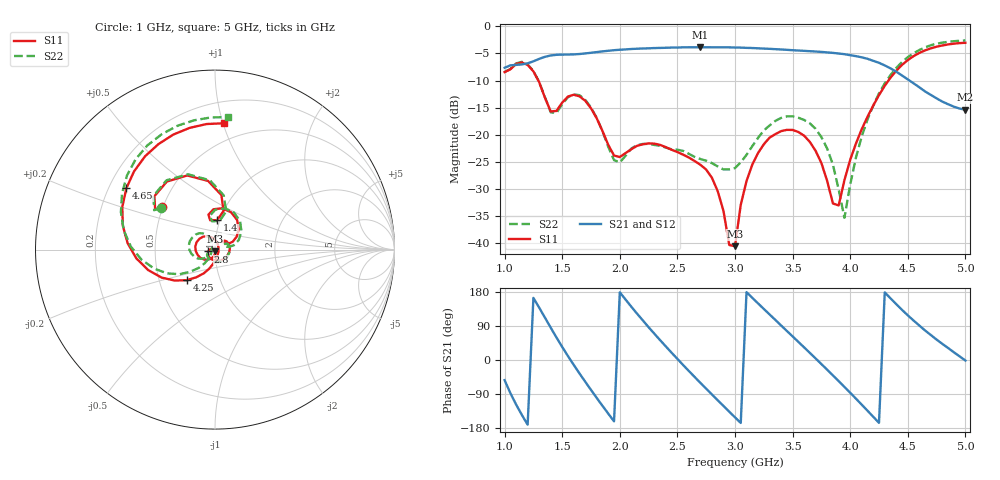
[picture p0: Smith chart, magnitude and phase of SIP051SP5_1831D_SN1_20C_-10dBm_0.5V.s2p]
# GHz  S  dB  R  50
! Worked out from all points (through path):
!   81 points, 1 GHz to 5 GHz, reference 50 ohm
!   highest |S21| = -3.84 dB at 2.7 GHz (marker M1); lowest = -15.4 dB at 5 GHz (marker M2)
!   lowest |S11| = -40.6 dB at 3 GHz (marker M3), VSWR 1.02, Z = 49.8 - j0.921 ohm
!   |S11| at or under -10 dB: 1.293 GHz to 4.332 GHz (3.04 GHz wide, 108 % of centre)
!   |S22| runs from -35.3 to -2.6 dB; largest |S21 - S12| = 0.0035
!   S11 on the Smith chart (normalised r, x): 1 GHz: 0.49, +0.27; 1.4 GHz: 0.97, +0.33; 2.8 GHz: 0.93, -0.02; 4.25 GHz: 0.69, -0.25; 4.65 GHz: 0.27, +0.29; 5 GHz: 0.36, +1.01
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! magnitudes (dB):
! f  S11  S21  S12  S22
! 1 GHz  -8.4  -7.6  -7.6  -8.4
! 1.2 GHz  -7.1  -6.8  -6.8  -7.0
! 1.4 GHz  -15.7  -5.4  -5.4  -15.8
! 1.7 GHz  -13.7  -5.0  -5.0  -13.5
! 1.95 GHz  -23.8  -4.4  -4.4  -24.7
! 2.35 GHz  -21.9  -4.0  -4.0  -22.0
! 2.7 GHz  -25.6  -3.8  -3.9  -24.5
! 2.8 GHz  -28.0  -3.9  -3.9  -25.2
! 2.95 GHz  -40.4  -3.9  -3.9  -26.4
! 3 GHz  -40.6  -3.9  -3.9  -26.2
! 3.1 GHz  -28.6  -4.0  -4.0  -23.7
! 3.25 GHz  -21.8  -4.1  -4.1  -19.2
! 3.5 GHz  -19.1  -4.4  -4.4  -16.6
! 3.7 GHz  -23.0  -4.6  -4.6  -18.9
! 3.85 GHz  -32.7  -4.9  -4.9  -25.5
! 3.9 GHz  -33.1  -5.0  -5.0  -30.1
! 3.95 GHz  -28.4  -5.1  -5.1  -35.3
! 4.1 GHz  -19.0  -5.7  -5.7  -20.3
! 4.25 GHz  -12.7  -6.7  -6.7  -12.4
! 4.35 GHz  -9.5  -7.7  -7.8  -9.0
! 4.65 GHz  -4.4  -12.0  -12.0  -3.9
! 5 GHz  -3.0  -15.4  -15.4  -2.6
